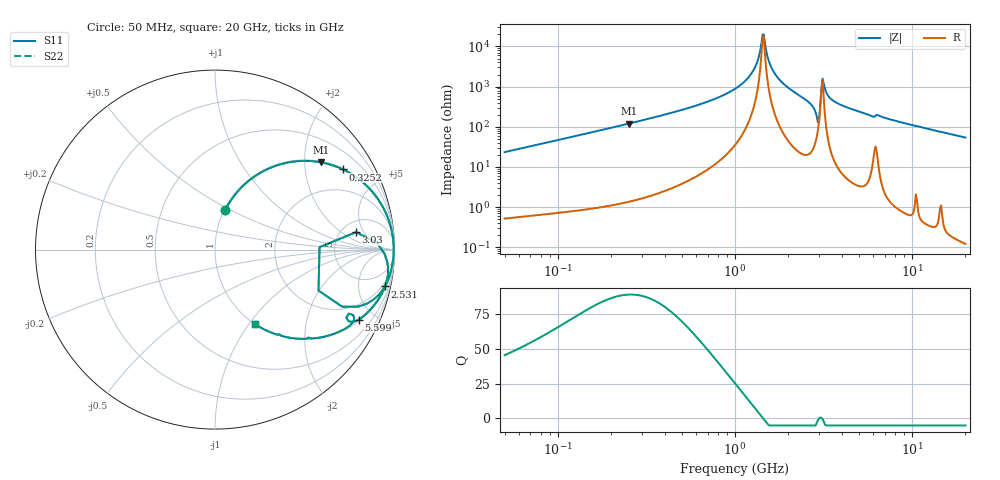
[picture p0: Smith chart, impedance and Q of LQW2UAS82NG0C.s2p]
!Murata Part Number: LQW2UAS82NG0C
!These Parameters are Measured in Series Mode Connection
!  o--[Z]--o
!Port1  Port2
!  o-------o
!Freq. Start=50[MHz] Stop=20[GHz], 401[Steps]
# Hz S RI R 50
!Freq.(Hz) S11(Real) S11(Imag) S21(Real) S21(Imag) S12(Real) S12(Imag) S22(Real) S22(Imag)
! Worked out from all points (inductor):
!   401 points, 50 MHz to 20 GHz, reference 50 ohm
!   read as one part in series: L = 74.2 nH near 51.52 MHz
!   highest Q = 88.6 at 252.1 MHz (marker M1), where L = 76 nH
!   self-resonance near 1.433 GHz
!   S11 on the Smith chart (normalised r, x): 50 MHz: 1.01, +0.47; 325.2 MHz: 1.04, +3.17; 2.531 GHz: 1.40, -9.11; 3.03 GHz: 6.75, +3.52; 5.599 GHz: 1.08, -4.07; 20 GHz: 1.00, -1.08
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5e7  0.0563 0.2197  0.9437 -0.2197  0.9437 -0.2197  0.0563 0.2197
1.364002e8  0.2921 0.4482  0.7079 -0.4482  0.7079 -0.4482  0.2921 0.4482
2.520729e8  0.5905 0.4861  0.4095 -0.4861  0.4095 -0.4861  0.5905 0.4861
3.251725e8  0.7128 0.4467  0.2872 -0.4467  0.2872 -0.4467  0.7128 0.4467
3.721004e8  0.7697 0.415  0.2303 -0.415  0.2303 -0.415  0.7697 0.415
6.774326e8  0.9372 0.2331  0.0628 -0.2331  0.0628 -0.2331  0.9372 0.2331
1e9  0.9829 0.1112  0.0171 -0.1112  0.0171 -0.1112  0.9829 0.1112
1.251922e9  0.9937 0.0431  0.00631 -0.0431  0.00631 -0.0431  0.9937 0.0431
1.329223e9  0.9949 0.025  0.00507 -0.025  0.00507 -0.025  0.9949 0.025
1.411297e9  0.9955 0.00682  0.00451 -0.00682  0.00451 -0.00682  0.9955 0.00682
1.454215e9  0.9955 -0.00231  0.00448 0.00231  0.00448 0.00231  0.9955 -0.00231
1.567309e9  0.9948 -0.0253  0.00516 0.0253  0.00516 0.0253  0.9948 -0.0253
1.714689e9  0.9925 -0.0536  0.00751 0.0536  0.00751 0.0536  0.9925 -0.0536
2.531158e9  0.946 -0.2053  0.054 0.2053  0.054 0.2053  0.946 -0.2053
2.728004e9  0.9004 -0.2637  0.0996 0.2637  0.0996 0.2637  0.9004 -0.2637
2.896447e9  0.7086 -0.3179  0.2914 0.3179  0.2914 0.3179  0.7086 -0.3179
3.029571e9  0.786 0.0972  0.214 -0.0972  0.214 -0.0972  0.786 0.0972
3.168813e9  0.96 -0.0696  0.04 0.0696  0.04 0.0696  0.96 -0.0696
3.626126e9  0.9424 -0.2168  0.0576 0.2168  0.0576 0.2168  0.9424 -0.2168
5.598765e9  0.8007 -0.3898  0.1993 0.3898  0.1993 0.3898  0.8007 -0.3898
7.442007e9  0.7035 -0.4522  0.2965 0.4522  0.2965 0.4522  0.7035 -0.4522
2e10  0.2256 -0.4168  0.7744 0.4168  0.7744 0.4168  0.2256 -0.4168
